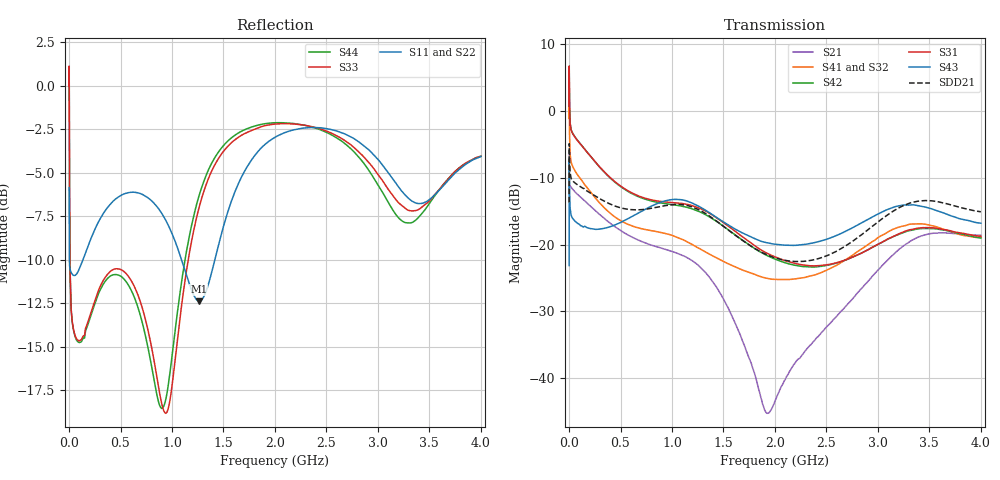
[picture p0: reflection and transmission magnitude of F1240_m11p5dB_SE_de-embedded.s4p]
! Integrated Device Technology
! Corporate Headquarters
! 6024 Silver Creek Valley Road
! San Jose, CA 95138  USA
! Phone:  1-408-284-8200
! Toll Free:  1-800-223-1366
! Webpage:  http://www.idt.com/
! Timing and RF Division
! 515 Groton Road, Suite 102
! Westford, MA 01886-6024
! Device:  F1240
! Description: Dual Intermediate Frequency Digital Variable Gain Amplifier
! Frequency:  10.0 -  500.00 MHz
! Package:  5x5 mm QFN Plastic Package: 32 pin
! Ports:  8 RF, 20 DC
!  Pin  1  = GA3 / Data  Pin 17  = RF OUT_B+
!  Pin  2  = GA4 / CLK  Pin 18  = RF OUT_B-
!  Pin  3  = GA5  Pin 19  = STBY_B
!  Pin  4  = VMODE  Pin 20  = Ground
!  Pin  5  = No Connect  Pin 21  = Ground
!  Pin  6  = GB5  Pin 22  = STB_A
!  Pin  7  = GB4  Pin 23  = RF OUT_A-  = Port 4
!  Pin  8  = GB3  Pin 24  = RF OUT_A+  = Port 3
!  Pin  9  = GB2  Pin 25  = GA0
!  Pin 10  = GB1  Pin 26  = ISET_A
!  Pin 11  = RF IN_B+  Pin 27  = VCC
!  Pin 12  = RF IN_B-  Pin 28  = Ground
!  Pin 13  = Ground  Pin 29  = RF IN_A-  = Port 2
!  Pin 14  = VCC  Pin 30  = RF IN_A+  = Port 1
!  Pin 15  = ISET_B  Pin 31  = GA1
!  Pin 16  = GB0  Pin 32  = GA2 / CSb
! Gain  = +19.5 dB
! State  = 1
! Voltage  = +5.00 V
! Current  = 85.292 mA (one channel only)
! Temperture  =  +25 C
! Test Date  =  2017-10-18
! Board  =  EB4031
! Data:  The device was measured on a custom evaluation board which has
!  individual transmission lines to the RF pins.  Data was collected
!  using a calibrated network analyzer.  The evaluation board was
!  de-embedded using Automatic Fixture Removal.
!  The reference plane is the edge of the package pin.
!  Only Channel A was measured.
!  This data is in single-ended operation.  If your needs are balanced
!  or differential S-parameters then this file needs to be used a
!  linear simulator.
! File Date:  2017-11-10  MJV
! Note:
!  Integrated Device Technology supplies this data as a sample of measured
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# Hz S dB R 100
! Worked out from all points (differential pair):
!   410 points, 500 kHz to 4 GHz, reference 100 ohm
!   strongest paths, dB at 500 kHz, 930 MHz, 1.96 GHz, 2.98 GHz, 4 GHz:
!     S43: -23.2, -13.5, -19.9, -15.6, -16.8
!     S31: 0.7, -13.6, -21.6, -20.1, -18.8
!     S42: 0.7, -13.9, -21.9, -20.2, -19.0
!     S41: -1.1, -18.3, -25.2, -19.2, -19.0
!     S32: -1.1, -18.5, -24.9, -19.4, -19.2
!     S21: -6.4, -20.7, -44.7, -24.2, -18.6
!   taken as a pair (ports 1,2 in; 3,4 out), SDD21 dB: -13.7, -14.2, -21.8, -16.9, -15.1
!   lowest |S11| = -12.4 dB at 1.26 GHz (marker M1), VSWR 1.63, Z = 61.9 - j8.49 ohm
!   |S11| at or under -10 dB: 3.335 MHz to 134.6 MHz (131.3 MHz wide, 190 % of centre); 1.093 GHz to 1.416 GHz (323 MHz wide, 25.8 % of centre)
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500000  -5.85 -5.6  -6.41 -5.8  -32.05 75.9  -33.83 75.3
        -6.42 -5.8  -5.85 -5.6  -33.79 74.1  -32.05 76.9
        0.68 -112.7  -1.13 -114.4  -0.01 -0.5  -23.16 -38.3
        -1.15 -113.2  0.68 -111.6  -23.15 -38.4  -0.02 1.8
3500000  -10.07 -15.6  -10.83 -14.6  -26.26 1.4  -29.97 -11.3
         -10.83 -14.6  -10.07 -15.7  -29.93 -11.6  -26.27 1.6
         2.29 153.2  -1.40 140.4  -4.21 -85.7  -9.80 173.6
         -1.42 140.7  2.29 153.4  -9.81 173.6  -4.25 -85.7
3.6e8  -7.10 -121.6  -16.34 -96.3  -31.34 -77.6  -37.44 -78.0
       -16.34 -96.3  -7.02 -122.3  -37.54 -76.3  -31.54 -77.5
       -9.41 61.2  -14.85 28.8  -10.93 -163.2  -17.57 50.7
       -14.78 28.0  -9.48 59.8  -17.52 50.3  -11.16 -164.0
1.26e9  -12.38 -164.4  -23.28 90.5  -30.48 123.5  -35.62 151.3
        -23.19 90.5  -12.22 -164.1  -35.42 154.5  -31.79 127.7
        -14.54 -134.6  -20.40 153.7  -7.06 -118.7  -14.43 169.6
        -20.55 146.4  -15.05 -135.7  -14.29 169.8  -6.36 -121.2
1.93e9  -3.23 -168.1  -44.87 38.1  -33.68 4.0  -36.42 24.3
        -45.23 34.7  -3.15 -168.6  -36.78 29.7  -35.03 11.1
        -21.35 88.3  -24.83 23.1  -2.26 -176.0  -19.96 50.0
        -25.07 16.6  -21.70 91.0  -19.75 50.9  -2.15 -179.0
3.23e9  -6.04 38.4  -20.37 -76.7  -26.70 145.1  -29.25 159.3
        -20.41 -76.7  -5.71 41.0  -29.39 173.4  -27.99 154.3
        -18.24 -127.5  -17.32 144.4  -6.87 23.2  -15.19 -159.0
        -17.28 130.5  -18.31 -124.0  -14.13 -158.3  -7.74 10.0
4e9  -4.06 -127.8  -18.61 125.6  -27.16 -17.0  -28.26 -2.3
     -18.62 125.7  -3.83 -126.3  -28.88 10.7  -28.85 -6.3
     -18.78 61.1  -19.19 -32.4  -4.05 -132.9  -18.20 61.2
     -18.96 -46.1  -19.03 67.1  -16.82 55.3  -4.05 -142.8
